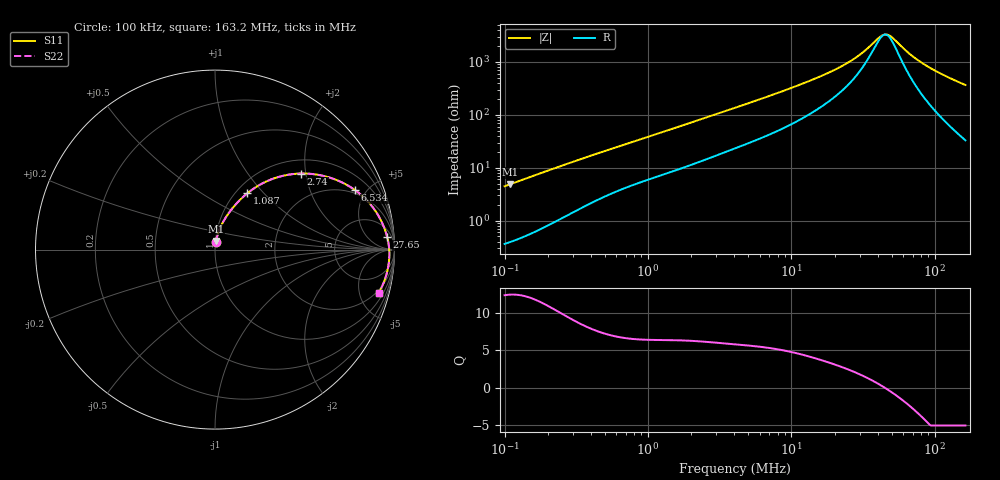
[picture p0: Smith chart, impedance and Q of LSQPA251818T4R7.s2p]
! LSQPA251818T4R7  S-PARAMETER MODEL  ( General Type )
! Model Generated by TAIYO YUDEN Corporation (http://www.ty-top.com)
! Version 3.0
! TAIYO YUDEN Control No. 160907NF25SB-FKC
! Copyright(c) 2007 TAIYO YUDEN CO.,LTD. All Rights Reserved.
! Product Description (link to TY-COMPAS)
! https://ds.yuden.co.jp/TYCOMPAS/or/detail?pn=LSQPA251818T4R7M&u=M
! Products Name : Inductors
! Characteristics :
!  Inductance : 4.7 uH , SRF(min) : 41 MHz , DC Resistance(max) : 0.26 Ohm
!  Rated Current : Saturation :680 mA , Temp Rise : 920 mA (40 degC)
!  Case Size : 2.5 x 1.8 / 0.098 x 0.071 [mm/inch] , Thickness : 1.8 / 0.071 [mm/inch]
!  (Conditions: Temperature = 25 degC , DC Bias Current/Voltage = 0A / 0V)
! External Node Assignments :
!  1  o---GGG---o  2
! GND o---------o GND
! Frequency Range : 0.1MHz  -  163.203978MHz  [ 402 STEP ]
# MHz S RI R 50
! Freq[MHz].  S11 Real  S11 Imag  S21 Real  S21 Imag  S12 Real  S12 Imag  S22 Real  S22 Imag
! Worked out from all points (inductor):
!   401 points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, 100 kHz to 163.2 MHz, reference 50 ohm
!   read as one part in series: L = 7.06 uH near 103.8 kHz
!   highest Q = 12.4 at 109.7 kHz (marker M1), where L = 7.07 uH
!   self-resonance near 44.86 MHz
!   S11 on the Smith chart (normalised r, x): 100 kHz: 1.01, +0.09; 1.087 MHz: 1.13, +0.82; 2.74 MHz: 1.31, +1.88; 6.534 MHz: 1.78, +4.19; 27.65 MHz: 11, +21; 163.2 MHz: 1.66, -7.32
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0.1  0.00556 0.0441  0.9944 -0.0441  0.9944 -0.0441  0.00556 0.0441
0.109688  0.00626 0.0482  0.9937 -0.0482  0.9937 -0.0482  0.00626 0.0482
0.345249  0.0372 0.1389  0.9628 -0.1389  0.9628 -0.1389  0.0372 0.1389
0.647462  0.093 0.2252  0.907 -0.2252  0.907 -0.2252  0.093 0.2252
1.08669  0.1804 0.3139  0.8196 -0.3139  0.8196 -0.3139  0.1804 0.3139
1.191969  0.2019 0.3303  0.7981 -0.3303  0.7981 -0.3303  0.2019 0.3303
1.892607  0.3403 0.4007  0.6597 -0.4007  0.6597 -0.4007  0.3403 0.4007
2.739662  0.4799 0.4239  0.5201 -0.4239  0.5201 -0.4239  0.4799 0.4239
4.115259  0.6352 0.4024  0.3648 -0.4024  0.3648 -0.4024  0.6352 0.4024
6.534207  0.7803 0.3314  0.2197 -0.3314  0.2197 -0.3314  0.7803 0.3314
9.458655  0.8607 0.2583  0.1393 -0.2583  0.1393 -0.2583  0.8607 0.2583
13.94754  0.9138 0.1831  0.0862 -0.1831  0.0862 -0.1831  0.9138 0.1831
20.56677  0.9449 0.1165  0.0551 -0.1165  0.0551 -0.1165  0.9449 0.1165
27.64874  0.9592 0.0709  0.0408 -0.0709  0.0408 -0.0709  0.9592 0.0709
32.05752  0.9642 0.0491  0.0358 -0.0491  0.0358 -0.0491  0.9642 0.0491
42.30653  0.97 0.00864  0.03 -0.00864  0.03 -0.00864  0.97 0.00864
45.55486  0.9709 -0.00226  0.0291 0.00226  0.0291 0.00226  0.9709 -0.00226
48.15376  0.9713 -0.0105  0.0287 0.0105  0.0287 0.0105  0.9713 -0.0105
67.17428  0.9698 -0.0623  0.0302 0.0623  0.0302 0.0623  0.9698 -0.0623
82.32906  0.965 -0.097  0.035 0.097  0.035 0.097  0.965 -0.097
112.7442  0.9496 -0.1574  0.0504 0.1574  0.0504 0.1574  0.9496 -0.1574
163.204  0.9124 -0.2413  0.0876 0.2413  0.0876 0.2413  0.9124 -0.2413
